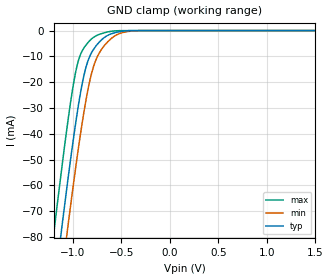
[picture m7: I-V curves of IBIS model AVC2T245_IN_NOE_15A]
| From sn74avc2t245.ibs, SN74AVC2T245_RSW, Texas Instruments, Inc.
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[Model]   AVC2T245_IN_NOE_15A
Model_type  Input
Vinl=0.49
Vinh=1.04
| variable   typ   min   max
C_comp   2.80pF   2.19pF   3.13pF
[Temperature Range]   40   100   -40
| Ambient temperature   25   85   -40
[Voltage range]   1.5   1.4   1.6
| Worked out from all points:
|   GND clamp passes 1 mA (typ) near -0.58 V on its own axis
[GND Clamp]
| AVC2T245_IN_NOE_15A
|   Voltage   I(typ)   I(min)   I(max)
-4.6V     -1.266A    -1.277A    -1.254A
-1.21V    -105.8mA   -124.1mA   -82.55mA
-1.185V   -97.95mA   -116.3mA   -74.69mA
-1.125V   -79.48mA   -97.82mA   -56.25mA
-1.06V    -60.14mA   -78.3mA    -37.34mA
-960mV    -32.94mA   -49.96mA   -14.03mA
-865mV    -14.14mA   -26.84mA   -5.576mA
-810mV    -8.703mA   -16.94mA   -3.298mA
-765mV    -6.095mA   -11.55mA   -2.106mA
-600mV    -1.191mA   -2.914mA   -255.1uA
-325mV    -4.51uA    -42.57uA   -26.57nA
1.5V      116.5pA    11.58nA    19.54pA
